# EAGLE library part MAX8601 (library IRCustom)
Maxim MAX8601 dual USB/DC lipoly battery charger http://www.ladyada.net/library/eagle
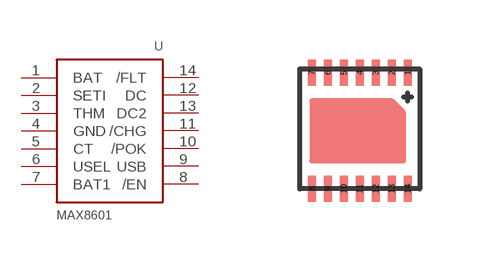
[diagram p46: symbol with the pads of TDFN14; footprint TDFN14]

Designator prefix -

## MAX8601  [TDFN14]
1  BAT  in
2  SETI  pas
3  THM  in
4  GND  pwr
5  CT  pas
6  USEL  in
7  BAT1  in
8  /EN  in
9  USB  in
10  /POK  out
11  /CHG  out
12  DC  in
13  DC2  in
14  /FLT  out

## Footprint TDFN14 (pad centres in mm)
smd 0.2 x 0.64: 1 1.2,1.4; 2 0.8,1.4; 3 0.4,1.4; 4 0,1.4; 5 -0.4,1.4; 6 -0.8,1.4; 7 -1.2,1.4; 8 -1.2,-1.5; 9 -0.8,-1.5; 10 -0.4,-1.5; 11 0,-1.5; 12 0.4,-1.5; 13 0.8,-1.5; 14 1.2,-1.5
